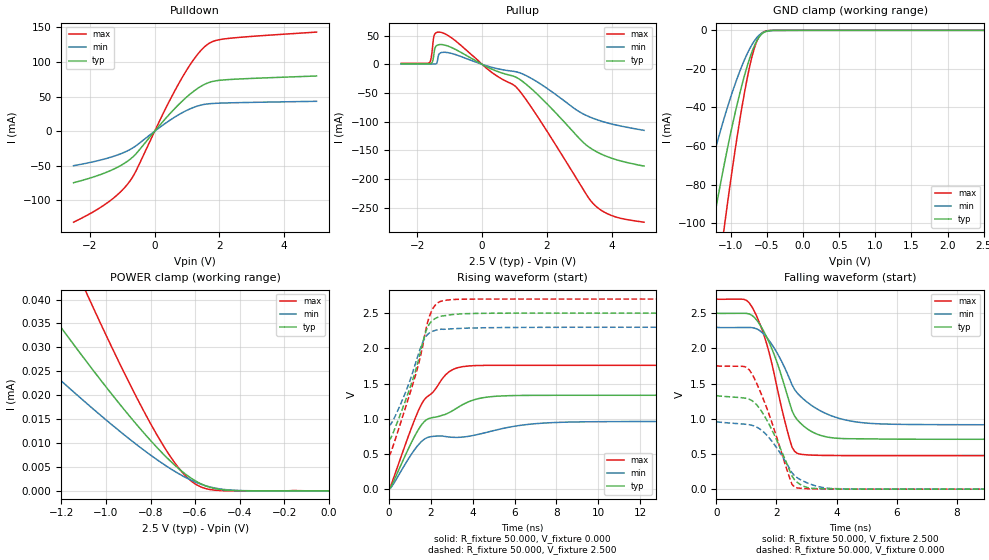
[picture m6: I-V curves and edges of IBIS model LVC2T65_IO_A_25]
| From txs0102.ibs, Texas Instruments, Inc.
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[Model]   LVC2T65_IO_A_25
Model_type  I/O
Vinl=0.15
Vinh=2.3
Enable   Active-High
Vref =   2.5
Rref =   1000000
Cref =   15p
Vmeas =   1.25
| variable   typ   min   max
C_comp   5.27pF   4.59pF   5.68pF
| C_pullup   6.03pF   4.57pF   7.36pF
| C_pulldown   5.97pF   5.23pF   7.08pF
| C_tri-state   5.27pF   4.59pF   5.68pF
[Temperature Range]   40   100   -40
| Ambient temperature   25   85   -40
[Voltage range]   2.5   2.3   2.7
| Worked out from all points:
|   slope of the pulldown table from 0 to 0.375 V, typ, clamps not added: 18.4 ohm
|   slope of the pullup table from 0 to 0.375 V, typ, clamps not added: 36.8 ohm
|   GND clamp passes 1 mA (typ) near -0.54 V on its own axis
|   rising waveform, R_fixture 50.000, V_fixture 0.000: 20-80 % time 2.24ns typ, 3.63ns min, 1.72ns max; typ from 0.003 V to 1.33 V
|   falling waveform, R_fixture 50.000, V_fixture 2.500: 20-80 % time 878ps typ, 1.29ns min, 778ps max; typ from 2.5 V to 0.709 V
|   rising waveform, R_fixture 50.000, V_fixture 2.500: 20-80 % time 1.13ns typ, 1.01ns min, 1.23ns max; typ from 0.694 V to 2.5 V
|   falling waveform, R_fixture 50.000, V_fixture 0.000: 20-80 % time 873ps typ, 922ps min, 848ps max; typ from 1.33 V to 0.003 V
[GND Clamp]
| LVC2T65_IO_A_25
|   Voltage   I(typ)   I(min)   I(max)
-2.5V     -423.2mA   -296.5mA   -584.2mA
-1.49V    -155.2mA   -103.2mA   -225.9mA
-1.44V    -143.5mA   -95.17mA   -209.4mA
-1.25V    -101.3mA   -66.57mA   -149.1mA
-1.1V     -71.12mA   -46.43mA   -104.7mA
-1.08V    -67.33mA   -43.92mA   -99mA
-910mV    -37.86mA   -24.61mA   -54.47mA
-765mV    -17.5mA    -11.48mA   -23.24mA
-705mV    -10.87mA   -7.264mA   -13.31mA
-650mV    -6.096mA   -4.225mA   -6.548mA
-545mV    -1.142mA   -915.6uA   -765.4uA
2.5V      253.4pA    2.854nA    61.17pA
[POWER Clamp]
| LVC2T65_IO_A_25
|   Voltage   I(typ)   I(min)   I(max)
-2.5V     124.2uA    82.51uA    202.8uA
-1.59V    59.69uA    39.88uA    95.71uA
-1.315V   41.43uA    27.82uA    65.33uA
-1.275V   38.85uA    26.12uA    61.03uA
-1.11V    28.43uA    19.25uA    43.69uA
-1.06V    25.36uA    17.23uA    38.6uA
-900mV    15.97uA    11.05uA    23uA
-760mV    8.542uA    6.177uA    10.83uA
-675mV    4.718uA    3.647uA    4.879uA
-615mV    2.575uA    2.189uA    1.979uA
-460mV    171.1nA    257.7nA    30.44nA
0V        0A         0A         0A
[Pulldown]
| LVC2T65_IO_A_25
|   Voltage   I(typ)   I(min)   I(max)
-2.5V     -74.46mA   -49.85mA   -131.4mA
-1.44V    -58.49mA   -38.81mA   -102.8mA
-1.085V   -50.62mA   -33.34mA   -89.19mA
-775mV    -41.27mA   -26.92mA   -73mA
-575mV    -32.73mA   -21.16mA   -57.59mA
230mV     12.46mA    7.881mA    22.14mA
760mV     39.18mA    24.2mA     69.92mA
1.2V      57.4mA     34.28mA    103mA
1.595V    68.75mA    39.12mA    124mA
1.805V    71.98mA    40.04mA    129.7mA
2.155V    74.13mA    40.72mA    133.3mA
5V        79.73mA    43.15mA    143.1mA
[Pullup]
| LVC2T65_IO_A_25
|   Voltage   I(typ)   I(min)   I(max)
-2.5V     981.5uA    517.1uA    1.69mA
-1.63V    1.061mA    502.1uA    2.617mA
-1.58V    1.394mA    502.5uA    8.593mA
-1.535V   3.987mA    505.3uA    26.3mA
-1.46V    27.03mA    543.5uA    52.74mA
-1.395V   32.9mA     2.47mA     55.7mA
-1.32V    34.42mA    18.42mA    56.26mA
-1.05V    31.83mA    20.43mA    50.33mA
1.09V     -23.75mA   -13.54mA   -41.94mA
3.475V    -150.8mA   -95.25mA   -245.8mA
4.12V     -166.1mA   -105.7mA   -266.4mA
5V        -177.7mA   -115.3mA   -275.6mA
[Ramp]
| LVC2T65_IO_A_25
| variable   typ   min   max
dV/dt_r   0.84/2.27E-09   0.61/3.67E-09   1.08/1.73E-09
dV/dt_f   1.07/8.75E-10   0.83/1.30E-09   1.33/7.78E-10
R_load = 50
[Rising Waveform]
R_fixture = 50.000
V_fixture = 0.000
V_fixture_min = 0.000
V_fixture_max = 0.000
C_fixture = 0.000
L_fixture = 0.000
|  time   V(typ)   V(min)   V(max)
0s        3.119mV    2.719mV    3.388mV
1.176ns   723.8mV    542.2mV    949.1mV
1.68ns    958.3mV    709.4mV    1.268V
2.184ns   1.023V     754mV      1.408V
2.94ns    1.099V     741.2mV    1.681V
3.864ns   1.25V      755.7mV    1.752V
4.536ns   1.302V     799.1mV    1.759V
7.14ns    1.334V     935.1mV    1.76V
12.01ns   1.335V     962.2mV    1.76V
419.9ns   1.33V      959mV      1.754V
[Falling Waveform]
R_fixture = 50.000
V_fixture = 2.500
V_fixture_min = 2.300
V_fixture_max = 2.700
C_fixture = 0.000
L_fixture = 0.000
|  time   V(typ)   V(min)   V(max)
0s        2.5V       2.3V       2.7V
1.092ns   2.489V     2.297V     2.646V
1.68ns    2.156V     2.154V     2.057V
2.016ns   1.805V     1.94V      1.455V
2.52ns    1.115V     1.482V     596.6mV
3.024ns   859.4mV    1.237V     489.4mV
3.696ns   742mV      1.067V     480.7mV
5.124ns   715.9mV    936.4mV    478.5mV
9.072ns   710.7mV    916.7mV    478.2mV
419.9ns   708.6mV    903.9mV    477.6mV
[Rising Waveform]
R_fixture = 50.000
V_fixture = 2.500
V_fixture_min = 2.300
V_fixture_max = 2.700
C_fixture = 0.000
L_fixture = 0.000
|  time   V(typ)   V(min)   V(max)
0s        694.4mV    903.9mV    470mV
336ps     901.2mV    1.062V     738mV
1.008ns   1.441V     1.547V     1.364V
1.344ns   1.757V     1.859V     1.698V
1.596ns   2.06V      2.074V     2.008V
1.848ns   2.301V     2.197V     2.372V
2.1ns     2.402V     2.245V     2.565V
2.52ns    2.459V     2.273V     2.672V
3.696ns   2.493V     2.287V     2.699V
419.9ns   2.5V       2.3V       2.7V
[Falling Waveform]
R_fixture = 50.000
V_fixture = 0.000
V_fixture_min = 0.000
V_fixture_max = 0.000
C_fixture = 0.000
L_fixture = 0.000
|  time   V(typ)   V(min)   V(max)
0s        1.33V      958.4mV    1.753V
924ps     1.296V     925.6mV    1.743V
1.092ns   1.279V     917.2mV    1.697V
1.344ns   1.198V     883mV      1.501V
1.68ns    981.8mV    767.8mV    1.151V
2.52ns    186.2mV    234.4mV    68.79mV
2.94ns    38.28mV    107.2mV    11.16mV
3.444ns   9.979mV    34.6mV     5.378mV
9.072ns   3.111mV    2.748mV    3.408mV
419.9ns   3.098mV    2.654mV    3.403mV
